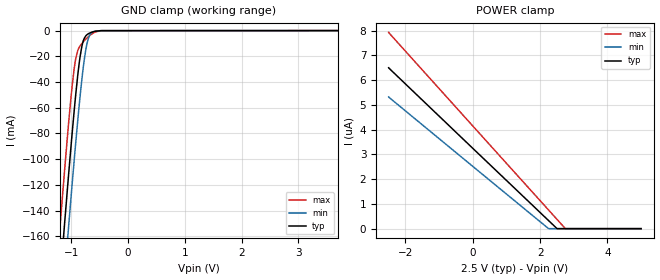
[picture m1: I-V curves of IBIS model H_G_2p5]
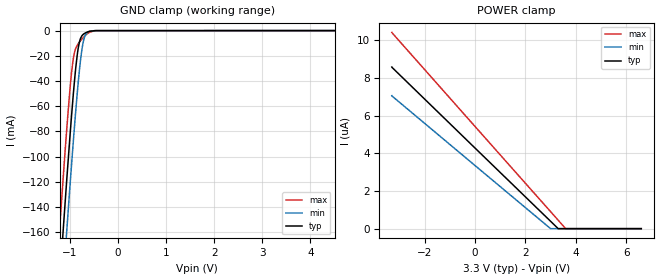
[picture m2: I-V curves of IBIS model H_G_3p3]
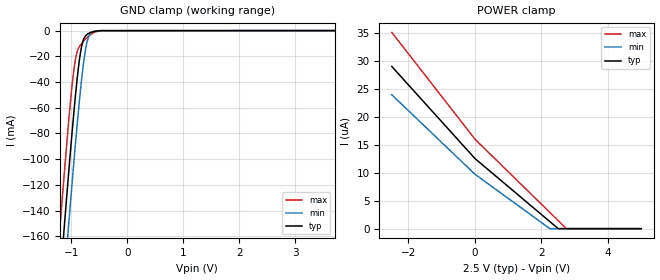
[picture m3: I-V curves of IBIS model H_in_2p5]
| Texas Instruments Incorporated
| 3.3V  LVCMOS High-Performance Clock Buffer
| Signal Rate: 200 kbps
| Marketing part#   Voltage Range   Package-type   #pins/pkg drawing
| cdclvc1110   2.25V - 3.6V   PW   20-pin TSSOP
[IBIS Ver]   4.1
[File name]   cdclvc1110.ibs
[File Rev]   1.0
[Date]   10/26/2010
[Source]   Model built from TISPICE simulations at:
   Texas Instruments Incorporated.
   Analog-eLab, HPA
   12500 TI Blvd
   Dallas, TX -75243
   For Support e-mail: elab_scm_ibis@list.ti.com
[Notes]   Revision History
   Rev 1.0: 08/02/2010
   - Model based on simulations from TIspiceD
   - C_comp values were obtained at 250MHz
   - For all buffers, Ccomp was obtained with the following corners:
   max C_comp was obtained at corner high VCC, low  temperature,
   strong process
   min C_comp was obtained at corner low  VCC, high temperature,
   weak process
   Rev 2.0: 10/26/2010
   - Appl. Eng. requested corrections for Vinh & Vinl
   In H_in_2p5 Vinh should be 1.65V.
   In H_in_3p3 Vinl should be 1.05V.
[Disclaimer] This product is designed as an aid for customers of Texas
   Instruments.
   No warranties, either expressed or implied, with respect
   to this third party software (if any) or with respect to
   its fitness for any particular purpose is claimed by Texas
   Instruments or the author. The software (if any) is provided
   solely on an "as is" basis. The entire risk as to its quality
   and performance is with the customer
[Copyright]   (C)Copyright 2010 Texas Instruments Incorporated.
   All rights reserved.
|   Component cvclvc1110pw
[Component]   cdclvc1110
[Manufacturer]  Texas Instruments Incorporated
[Package]   |20-pin TSSOP package
|   typ   min   max
R_pkg   0.19391   0.11447   0.22353
L_pkg   3.02017nH   2.49185nH   3.49527nH
C_pkg   0.51850pF   0.43419pF   0.61010pF
[Pin] signal_name   model_name   R_pin   L_pin   C_pin
1   CLKIN   H_in   0.18678 3.47583nH 0.60907pF
2   1G   H_G   0.19559 3.18028nH 0.57784pF
3   Y0   H_out   0.21769 3.09158nH 0.49262pF
4   GND   GND   0.19544 2.71074nH 0.44812pF
5   VDD   POWER   0.18740 2.64378nH 0.43486pF
6   Y4   H_out   0.18811 2.65174nH 0.43730pF
7   GND   GND   0.20212 2.78000nH 0.45303pF
8   Y6   H_out   0.22353 3.15835nH 0.49762pF
9   VDD   POWER   0.20673 3.31417nH 0.59227pF
10   Y9   H_out   0.18797 3.49527nH 0.60829pF
11   GND   GND   0.18799 3.49480nH 0.61010pF
12   Y8   H_out   0.20580 3.30300nH 0.59404pF
13   Y7   H_out   0.22346 3.15448nH 0.49846pF
14   VDD   POWER   0.20212 2.78007nH 0.45283pF
15   Y5   H_out   0.18812 2.65200nH 0.43515pF
16   GND   GND   0.18641 2.63441nH 0.43419pF
17   Y2   H_out   0.19544 2.71072nH 0.45116pF
18   VDD   POWER   0.11447 2.49185nH 0.54952pF
19   Y3   H_out   0.19608 3.20248nH 0.58566pF
20   Y1   H_out   0.18692 3.47786nH 0.60793pF
[Pin Mapping]pulldown_ref pullup_ref gnd_clamp_ref power_clamp_ref |ext_ref
 1   NC   NC   GNDBUS   PWRBUS   | CLKIN
 2   NC   NC   GNDBUS   PWRBUS   | 1G
 3   GNDBUS   PWRBUS   NC   NC   | Y0
 4   GNDBUS   NC   | GND
 5   NC   PWRBUS   | VDD
 6   GNDBUS   PWRBUS   NC   NC   | Y4
 7   GNDBUS   NC   | GND
 8   GNDBUS   PWRBUS   NC   NC   | Y6
 9   NC   PWRBUS   | VDD
10   GNDBUS   PWRBUS   NC   NC   | Y9
11   GNDBUS   NC   | GND
12   GNDBUS   PWRBUS   NC   NC   | Y8
13   GNDBUS   PWRBUS   NC   NC   | Y7
14   NC   PWRBUS   | VDD
15   GNDBUS   PWRBUS   NC   NC   | Y5
16   GNDBUS   NC   | GND
17   GNDBUS   PWRBUS   NC   NC   | Y2
18   NC   PWRBUS   | VDD
19   GNDBUS   PWRBUS   NC   NC   | Y3
20   GNDBUS   PWRBUS   NC   NC   | Y1
[Model Selector] H_G
H_G_2p5   H_G Input model  at 2.5V
H_G_3p3   H_G Input model  at 3.3V
[Model Selector] H_in
H_in_2p5   H_in Input model at 2.5V
H_in_3p3   H_in Input model at 3.3V
[Model Selector] H_out
H_out_2p5   H_out Output model at 2.5V
H_out_3p3   H_out Output model at 3.3V
| Models and submodels in the file (6): H_G_2p5 (Input), H_G_3p3 (Input), H_in_2p5 (Input), H_in_3p3 (Input), H_out_2p5 (Output), H_out_3p3 (Output)
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|   H_G_2p5
[Model]   H_G_2p5
|Signal:   1G
Model_type   Input
Vinl   = 0.85
Vinh   = 1.65
|   typ   min   max
C_comp   910fF   809fF   967fF
[Voltage Range]   2.5   2.25   2.75
[Temperature Range]   25   85   -40
[Power Clamp Reference]   2.5   2.25   2.75
[GND Clamp Reference]   0   0   0
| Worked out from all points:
|   GND clamp passes 1 mA (typ) near -0.62 V on its own axis
[GND Clamp]
|   Voltage   I(typ)   I(min)   I(max)
-2.5V     -968.1mA   -1.007A    -929mA
-1.21V    -199mA     -240.4mA   -156.9mA
-1.15V    -165.5mA   -206.8mA   -123.9mA
-1.12V    -149.1mA   -190.2mA   -107.7mA
-1.064V   -118.8mA   -159.4mA   -78.45mA
-1.045V   -108.9mA   -149.3mA   -69.13mA
-947.5mV  -60.05mA   -98.34mA   -28.07mA
-850mV    -20.81mA   -51.87mA   -12.03mA
-771.2mV  -5.755mA   -21.65mA   -7.739mA
-681.3mV  -1.974mA   -3.841mA   -3.953mA
-463.7mV  -54uA      -32.29uA   -94.42uA
5V        0A         0A         0A
[POWER Clamp]
|   Voltage   I(typ)   I(min)   I(max)
-2.5V     6.5uA      5.321uA    7.929uA
2.251V    325.7nA    0A         752.1nA
2.502V    0A         0A         373.2nA
2.75V     0A         0A         0A
5V        0A         0A         0A
|   H_G_3p3
[Model]   H_G_3p3
|Signal:   1G
Model_type   Input
Vinl   = 1.05
Vinh   = 2.25
|   typ   min   max
C_comp   831.2f   785f   940.5f
[Voltage Range]   3.3   3   3.6
[Temperature Range]   25   85   -40
[Power Clamp Reference]   3.3   3   3.6
[GND Clamp Reference]   0   0   0
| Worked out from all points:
|   GND clamp passes 1 mA (typ) near -0.62 V on its own axis
[GND Clamp]
|   Voltage   I(typ)   I(min)   I(max)
-3.3V     -1.461A    -1.498A    -1.424A
-1.221V   -205.1mA   -246.6mA   -163.1mA
-1.206V   -196.8mA   -238.2mA   -154.8mA
-1.137V   -158.3mA   -199.5mA   -116.7mA
-1.063V   -118.2mA   -158.8mA   -77.87mA
-993.3mV  -82.31mA   -121.9mA   -45.27mA
-933.9mV  -53.76mA   -91.51mA   -24.11mA
-834.9mV  -16.5mA    -45.37mA   -11.07mA
-790.3mV  -7.806mA   -28.02mA   -8.666mA
-730.9mV  -3.374mA   -11.05mA   -5.922mA
-632mV    -1.127mA   -1.236mA   -2.355mA
6.6V      0A         0A         0A
[POWER Clamp]
|   Voltage   I(typ)   I(min)   I(max)
-3.3V     8.58uA     7.058uA    10.42uA
3.001V    391.5nA    0A         903.2nA
3.303V    0A         0A         447.8nA
3.6V      0A         0A         0A
6.6V      0A         0A         0A
|   H_in_2p5
[Model]   H_in_2p5
|Signal:   CLK_IN
Model_type   Input
Vinl   = 0.85
Vinh   = 1.65
|   typ   min   max
C_comp   0.943pF   0.765pF   1.207pF
[Voltage Range]   2.5   2.25   2.75
[Temperature Range]   25   85   -40
[Power Clamp Reference]   2.5   2.25   2.75
[GND Clamp Reference]   0   0   0
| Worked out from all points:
|   GND clamp passes 1 mA (typ) near -0.62 V on its own axis
[GND Clamp]
|   Voltage   I(typ)   I(min)   I(max)
-2.5V     -968.1mA   -1.007A    -929mA
-1.21V    -199mA     -240.4mA   -156.9mA
-1.15V    -165.6mA   -206.8mA   -123.9mA
-1.12V    -149.1mA   -190.2mA   -107.7mA
-1.064V   -118.8mA   -159.4mA   -78.47mA
-1.045V   -108.9mA   -149.3mA   -69.14mA
-947.5mV  -60.06mA   -98.34mA   -28.08mA
-850mV    -20.82mA   -51.87mA   -12.04mA
-771.2mV  -5.763mA   -21.66mA   -7.749mA
-681.3mV  -1.981mA   -3.847mA   -3.963mA
-463.7mV  -60.38uA   -37.46uA   -102.3uA
5V        0A         0A         0A
[POWER Clamp]
|   Voltage   I(typ)   I(min)   I(max)
-2.5V     29.05uA    23.98uA    35.15uA
1.25mV    12.55uA    9.742uA    16.01uA
2.251V    1.261uA    0A         2.905uA
2.502V    0A         0A         1.442uA
2.75V     0A         0A         0A
5V        0A         0A         0A
